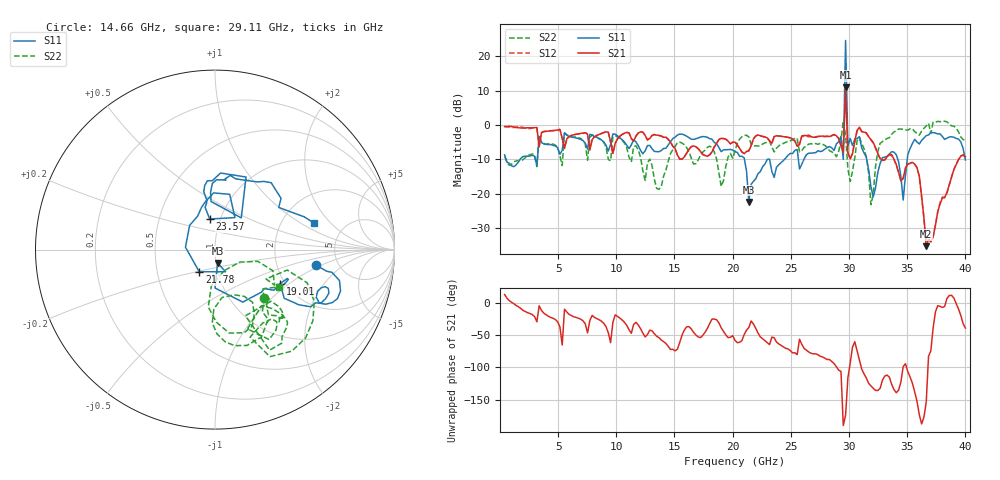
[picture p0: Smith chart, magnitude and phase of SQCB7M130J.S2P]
! Network Analyzer HP8722ES.07.66: Jul 25, 2000 Serial No. US39175408
! 26 Oct 2004  16:11:04
! Frequency  S11  S21  S12  S22
# HZ  S  DB R  50
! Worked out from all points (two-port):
!   201 points, 400 MHz to 40 GHz, reference 50 ohm
!   highest |S21| = 11.02 dB at 29.7 GHz (marker M1); lowest = -35.3 dB at 36.63 GHz (marker M2)
!   |S21| within 3 dB of the highest: 29.67259 GHz to 29.73507 GHz (62.48 MHz wide, 0.21 % of centre)
!   lowest |S11| = -22.4 dB at 21.39 GHz (marker M3), VSWR 1.16, Z = 50.9 - j7.62 ohm
!   |S11| at or under -10 dB: 523.3 MHz to 1.734 GHz (1.211 GHz wide, 107 % of centre); 21.01 GHz to 22.99 GHz (1.975 GHz wide, 8.98 % of centre); 23.17 GHz to 24.46 GHz (1.284 GHz wide, 5.39 % of centre)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
!   |S22| runs from -23.2 to 1.2 dB; largest |S21 - S12| = 2.5
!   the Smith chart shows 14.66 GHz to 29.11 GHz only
!   S11 on the Smith chart (normalised r, x): 14.66 GHz: 3.41, -0.87; 19.01 GHz: 1.88, -0.86; 21.78 GHz: 0.82, -0.21; 23.57 GHz: 0.89, +0.31; 29.11 GHz: 3.00, +1.32
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4e8  -8.69 -80.2  -0.48 12.7  -0.35 14.9  -9.11 -74.8
7.132e9  -4.57 -92.6  -2.37 -27.8  -2.45 -28.5  -4.56 -141.0
1.3666e10  -7.78 -30.3  -3.06 -53.9  -3.04 -53.8  -18.72 -93.1
1.4656e10  -4.88 -8.7  -4.97 -72.1  -4.92 -72.0  -8.32 -44.5
1.9012e10  -7.76 -27.5  -3.88 -38.7  -3.90 -38.7  -17.87 -66.3
2.02e10  -7.76 -28.9  -4.99 -58.1  -4.89 -57.3  -7.57 -15.8
2.1388e10  -22.40 -78.9  -7.52 -38.4  -7.51 -37.8  -3.47 -62.8
2.1784e10  -16.40 -125.4  -4.09 -32.8  -4.09 -31.7  -6.25 -56.7
2.3566e10  -15.24 99.9  -3.36 -54.2  -3.31 -53.3  -7.83 -50.4
2.6932e10  -8.12 81.1  -3.58 -79.0  -3.51 -80.8  -5.67 -44.9
2.911e10  -4.89 15.2  -3.96 -104.0  -3.82 -104.8  -7.70 -30.3
2.9506e10  -10.00 0.3  -7.89 170.5  -6.89 -123.1  1.19 60.2
2.9704e10  24.61 -82.5  11.02 -173.6  10.74 -131.4  -2.97 167.0
2.9902e10  -6.15 -116.8  -8.10 -116.1  -8.15 -114.9  -12.80 -64.9
3.0496e10  -4.12 -102.0  -4.74 -60.2  -4.80 -60.4  -9.49 -7.0
3.0694e10  -3.95 43.1  -1.55 -74.3  -1.65 -74.6  -4.57 160.2
3.1882e10  -17.98 117.3  -4.25 -128.4  -4.37 -128.8  -23.21 -128.1
3.3466e10  -8.45 -97.7  -8.49 -115.0  -8.69 -115.8  -3.71 23.8
3.4654e10  -21.85 -99.8  -15.58 -98.5  -15.52 -96.4  -1.30 7.6
3.5842e10  -4.96 -90.6  -12.39 -152.2  -12.39 -153.1  -2.44 9.0
3.6634e10  -3.10 -93.5  -35.28 -153.5  -35.19 -154.4  -0.26 22.8
4e10  -10.20 -125.9  -9.26 -39.1  -9.26 -38.8  -4.44 -23.3
